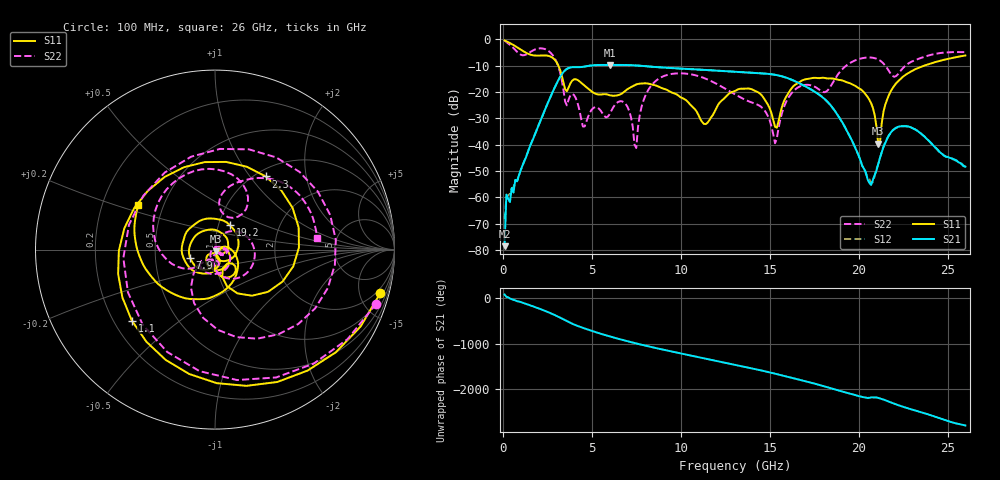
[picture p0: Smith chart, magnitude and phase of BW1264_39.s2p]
!Keysight Technologies,N5245B,MY57181159,A.13.60.06
!Date: Friday, December 18, 2020 23:54:06
!Correction: S11(Full 2 Port(1,2))
!S21(Full 2 Port(1,2))
!S12(Full 2 Port(1,2))
!S22(Full 2 Port(1,2))
!S2P File: Measurements: S11, S21, S12, S22:
# Hz S  dB  R 50
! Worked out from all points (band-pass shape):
!   260 points, 100 MHz to 26 GHz, reference 50 ohm
!   highest |S21| = -9.71 dB at 6 GHz (marker M1); lowest = -78.6 dB at 100 MHz (marker M2)
!   |S21| within 3 dB of the highest: 3.375 GHz to 14.04 GHz (10.66 GHz wide, 122 % of centre)
!   lowest |S11| = -39.6 dB at 21.1 GHz (marker M3), VSWR 1.02, Z = 50.5 - j0.947 ohm
!   |S11| at or under -10 dB: 3.123 GHz to 23.68 GHz (20.55 GHz wide, 153 % of centre)
!   |S22| runs from -41.3 to -0.5 dB; largest |S21 - S12| = 0.00063
!   S11 on the Smith chart (normalised r, x): 100 MHz: 1.42, -7.43; 1.1 GHz: 0.27, -0.34; 2.3 GHz: 1.11, +1.20; 7.9 GHz: 0.75, -0.07; 19.2 GHz: 1.13, +0.32; 26 GHz: 0.36, +0.23
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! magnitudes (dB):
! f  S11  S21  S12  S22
! 100 MHz  -0.4  -78.6  -68.3  -0.5
! 200 MHz  -0.7  -58.9  -59.9  -1.0
! 1.1 GHz  -4.3  -48.0  -48.2  -6.0
! 2.3 GHz  -6.1  -27.8  -27.8  -3.6
! 3.6 GHz  -19.7  -11.2  -11.2  -25.1
! 4.5 GHz  -17.1  -10.4  -10.4  -33.1
! 6 GHz  -21.2  -9.7  -9.7  -28.5
! 6.9 GHz  -19.5  -9.7  -9.7  -24.5
! 7.5 GHz  -17.1  -9.9  -9.9  -41.3
! 7.9 GHz  -16.7  -10.1  -10.1  -23.3
! 8.8 GHz  -18.1  -10.6  -10.6  -14.8
! 11.4 GHz  -32.2  -11.6  -11.6  -14.9
! 13.1 GHz  -19.4  -12.3  -12.3  -21.0
! 14.7 GHz  -22.7  -13.0  -13.0  -26.9
! 15.3 GHz  -33.2  -13.5  -13.5  -39.5
! 16.1 GHz  -19.9  -15.0  -15.0  -21.6
! 17.4 GHz  -14.7  -19.4  -19.3  -17.6
! 19.2 GHz  -15.9  -33.0  -33.0  -10.6
! 20.7 GHz  -24.3  -55.3  -54.7  -6.9
! 21.1 GHz  -39.6  -47.4  -47.4  -7.6
! 21.7 GHz  -21.2  -36.5  -36.5  -12.0
! 26 GHz  -6.1  -48.3  -48.4  -4.9
